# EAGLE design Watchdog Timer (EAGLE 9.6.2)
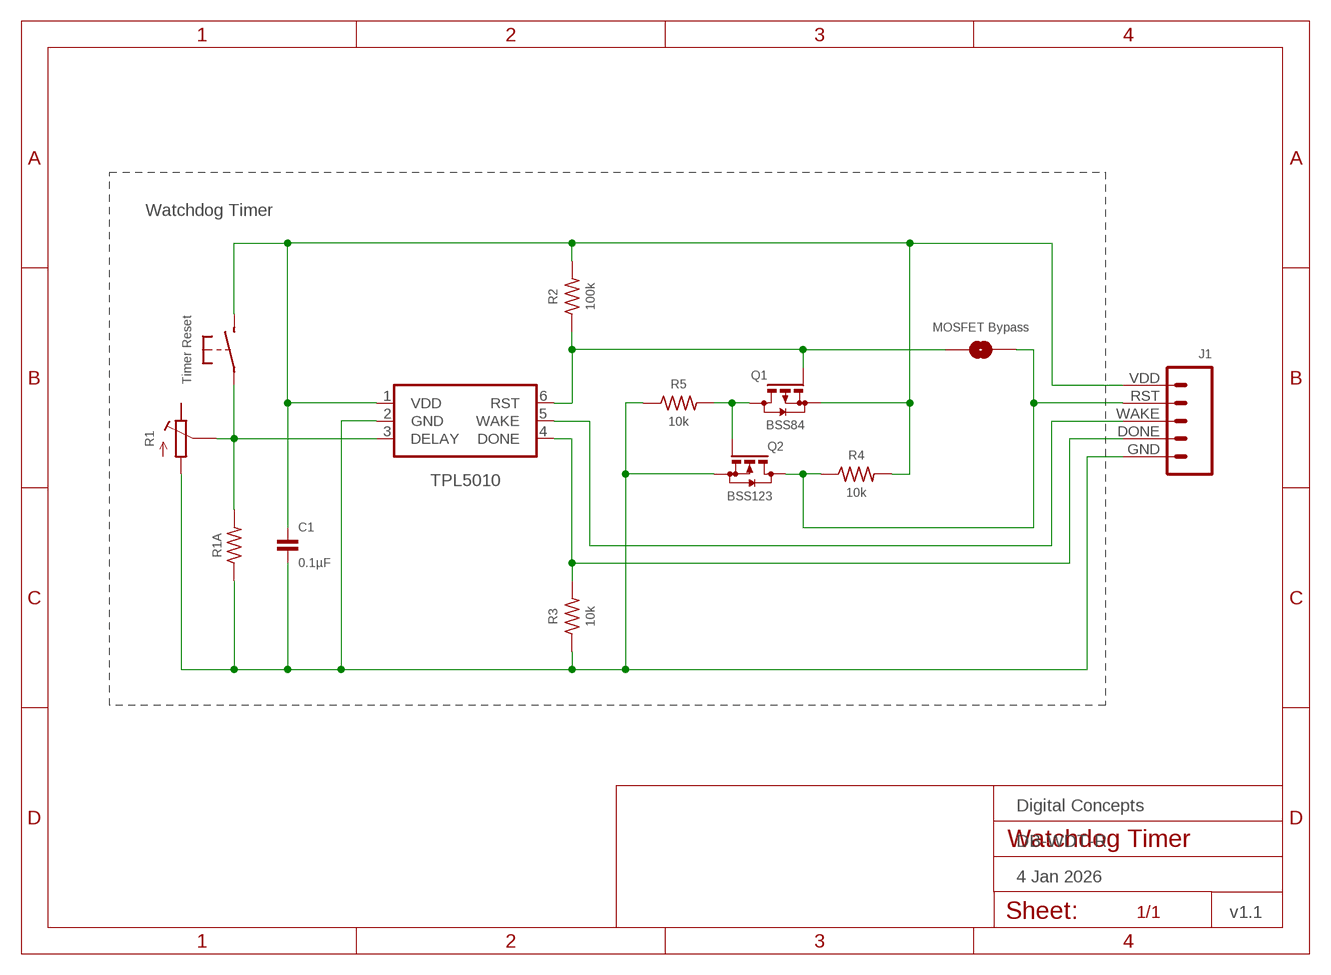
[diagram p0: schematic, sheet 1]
FRAME1 (FRAME_A5L-LOC): DATE: 4 Jan 2026; OWNER: Digital Concepts; TITLE: DB-WDT-R; VERSION: v1.1

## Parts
C1  0.1µF  CAPACITOR-0603  [C0603]
J1  HEADER-1X5-WDT  [CONN_05-WDT]
Q1  BSS84  MOSFET-BSS84  [SOT23-3]
Q2  BSS123  MOSFET-BSS123  [SOT23-3]
R1  RESISTOR-TRIMM-33  [RTRIM3*3]
R1A  RESISTOR-0603  [R0603]
R2  100k  RESISTOR-0603  [R0603]
R3  10k  RESISTOR-0603  [R0603]
R4  10k  RESISTOR-0603  [R0603]
R5  10k  RESISTOR-0603  [R0603]
S1  Timer Reset  SWITCH-MOMENTARY-2-PIN  [SWITCH-2-PAD]
SJ  MOSFET Bypass  SJ-V-2  [SJ-VIA-2]
U1  TPL5010  TPL5010DDCR  [SOT-23-6]

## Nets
GND: C1.2 J1.GND Q2.2(S) R1.1(A) R1A.1 R3.1 R5.1 U1.2(GND)
N$1: Q1.1(G) R2.1 SJ.1 U1.6(RST)
N$2: J1.WAKE U1.5(WAKE)
N$14: C1.1 J1.VDD Q1.2(S) R2.2 R4.2 S1.P$2(S) U1.1(VDD)
N$35: J1.RST Q2.3(D) R4.1 SJ.2 SJ.2@V
N$36: R1.2(S) R1A.2 S1.P$1(P) U1.3(DELAY)
N$38: J1.DONE R3.2 U1.4(DONE)
N$43: Q1.3(D) Q2.1(G) R5.2
Unconnected: R1.3(E)

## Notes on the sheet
- Watchdog Timer

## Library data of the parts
C1 = digitalconcepts:CAPACITOR-0603: 0603 Capacitor
J1 = digitalconcepts:HEADER-1X5-WDT: Single Row 5-Pin Header
Q1 = digitalconcepts:MOSFET-BSS84: P-CHANNEL MOS FET
Q2 = digitalconcepts:MOSFET-BSS123: N-CHANNEL MOS FET
R1 = digitalconcepts:RESISTOR-TRIMM-3*3: Trimm Resistor - 3*3 SMD
R1A R2-R5 = digitalconcepts:RESISTOR-0603: Resistor
S1 = digitalconcepts:SWITCH-MOMENTARY-2-PIN: 2 Pin Momentary Switch
SJ = digitalconcepts:SJ-V-2: Solder Jumper with Pad Vias
U1 = digitalconcepts:TPL5010DDCR: TPL5010 Nano-Power System Timer with Watchdog

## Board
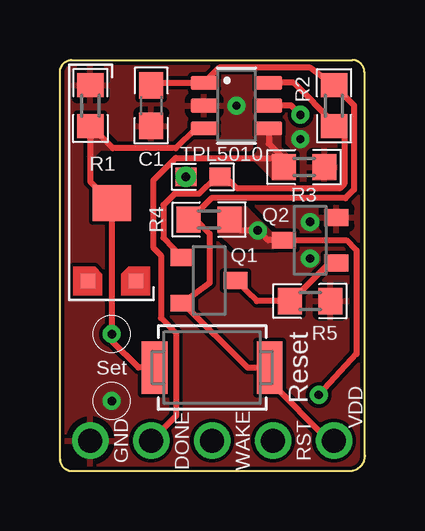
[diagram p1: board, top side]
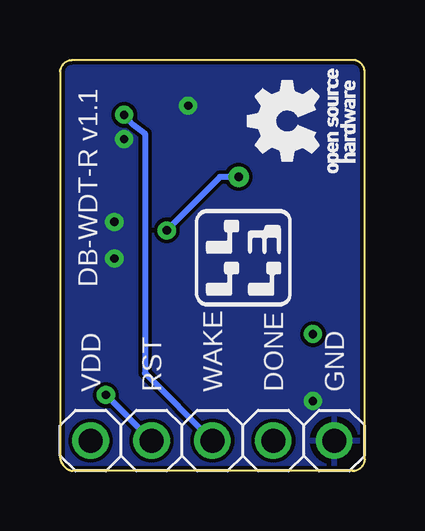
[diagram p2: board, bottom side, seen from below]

Size 12.71 x 17.15 mm. Coordinates in mm from the lower left corner, seen from the top.
Outline: 12.7,0.51 12.7,16.64 arc90 12.19,17.15 0.51,17.15 arc90 0,16.64 0,0.51 arc90 0.51,0 12.19,0 arc67 12.7,0.51
Outline: 12.7,0.76 arc-23 12.7,0.51
Copper layers (1*16): Top 0.035mm / dielectric 1.5mm / Bottom 0.035mm
Design rules "default *": minimum track width 6mil, minimum drill 0.35mm, track to track 6mil, track to pad 6mil, pad to pad 6mil, via to via 6mil, smd to smd 6mil, copper to edge 6mil, drill to drill 6mil, minimum pad ring 10mil, minimum via ring 8mil, stop-mask expansion 4mil, vias tented up to drill 0mil, thermal gap 10mil

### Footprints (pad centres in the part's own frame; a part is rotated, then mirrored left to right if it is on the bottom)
C0603 = smd 1.1 x 1: 1 -0.85,0; 2 0.85,0
CONN_05-WDT = drill 1 pad 1.524: DONE 2.54,0; GND 0,0; RST 7.62,0; VDD 10.16,0; WAKE 5.08,0
SOT23-3 = smd 0.7 x 1: 1 -0.95,-1.1; 2 0.95,-1.1; 3 0,1.1
RTRIM3*3 = smd 0.6 x 0.6: 1 -1,-1.6; 3 1,-1.6 | smd 1.6 x 1.5: 2 0,1.65
R0603 = smd 1 x 1.1: 1 -0.85,0; 2 0.85,0
SWITCH-2-PAD = smd 1.067 x 2.184: P$1 -2.4,0; P$2 2.4,0
SJ-VIA-2 = smd 0.864 x 0.762: 1 -0.711,0; 2 0.711,0 | drill 0.35 pad 0.61: 2@V 0.711,0
SOT-23-6 = smd 1.1 x 0.6: 1 -1.35,0.95; 2 -1.35,0; 3 -1.35,-0.95; 4 1.35,-0.95; 5 1.35,0; 6 1.35,0.95

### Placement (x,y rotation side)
C1  3.81,15.24 270 top
J1  1.27,1.27 180 bottom
Q1  6.22,7.95 270 top
Q2  10.44,9.63 90 top
R1  2.16,9.52 0 top
R1A  1.27,15.24 270 top
R2  11.43,15.24 90 top
R3  10.19,12.67 180 top
R4  6.22,10.49 180 top
R5  10.44,7.09 180 top
S1  6.35,4.32 0 top
SJ  5.97,12.27 180 top
U1  7.37,15.24 0 top

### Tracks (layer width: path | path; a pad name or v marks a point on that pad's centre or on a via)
GND  (via drill 0.35)
  other vias: 10.44,10.39 10.44,8.86 7.37,15.24 2.16,2.92 10.03,13.84
  pour Top (rank 5): -0.61,17.78 13.36,17.78 13.36,-0.63 -0.61,-0.63
  pour Bottom: -0.36,17.55 13.08,17.55 13.08,-0.38 -0.36,-0.38
N$1
  Top 0.254: U1.6 9.76,16.19 11.43,14.52 R2.1 11.86,13.96 11.86,11.98 11.67,11.79 7.39,11.79 6.91,12.27 SJ.1 6.5,12.27 5.79,11.56 4.77,11.56 4.32,11.1 4.32,9.73 Q1.1
N$2  (via drill 0.35)
  Top 0.254: v10.03,14.86 9.65,15.24 U1.5
  Bottom 0.254: v10.03,14.86 9.65,14.44 9.17,14.07 9.17,4.09 J1.WAKE
N$14
  Top 0.254: C1.1 4.29,16.19 U1.1 6.64,16.81 10.45,16.81 R2.2 12.27,15.25 12.27,11.73 11.91,11.38 6.31,11.38 5.42,10.49 R4.2 5.65,10.49 6.25,9.89 6.25,7.85 Q1.2 7.83,4.32 S1.P$2 8.75,3.75 11.23,1.27 J1.VDD
N$35  (via drill 0.35)
  Top 0.254: v10.8,3.18 12.37,4.88 12.37,9.2 11.94,9.63 Q2.3 8.69,9.63 v8.26,10.03 7.53,10.03 R4.1
  Bottom 0.254: v10.8,3.18 J1.RST | v8.26,10.03 6.05,12.27 SJ.2@V
  pour Top (no thermals): 6.6,9.96 7.26,9.3 8.91,9.3 9.34,9.45 7.8,11 6.6,11
N$36  (via drill 0.35)
  Top 0.254: U1.3 5.66,14.29 4.83,13.46 2.2,13.46 R1A.2 1.27,12.06 R1.2 v2.16,5.71 2.16,5.44 3.28,4.32 S1.P$1
  pour Top (rank 3, no thermals): 1.27,14.4 2.21,13.46 1.65,13.46 1.27,13.08
N$38
  Top 0.254: J1.DONE 4.85,2.31 4.85,5.74 4.22,6.38 4.22,9 3.89,9.33 3.89,12.12 4.83,13.06 8.95,13.06 R3.2 9.34,13.04 8.72,13.66 U1.4
  pour Top: 9.7,13.18 9.78,13.18 9.78,12.17 8.94,12.17 8.86,12.24 8.86,12.62
  pour Top (no thermals): 8.23,14.07 8.23,13.31 7.99,13.07 8.89,12.17 9.58,12.17 9.73,12.32 9.73,12.98 9.22,13.49 9.22,14.07
N$43
  Top 0.254: Q1.3 8.21,7.09 R5.2 9.67,7.09 11.2,8.63 11.49,8.63 Q2.1

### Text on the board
tPlace: Set | Reset | VDD | GND | DONE | WAKE | RST
bPlace: DB-WDT-R v1.1
bNames: GND | DONE | WAKE | RST | VDD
